FUNCTION_BLOCK FB_SignalHandlingDelay EXTENDS FB_SignalHandling
VAR_INPUT
	tiDelay			: TIME;
END_VAR
VAR
	bSet			: BOOL;
	tonDelay		: TON;
END_VAR

// =========================================================
;
// =========================================================

METHOD PUBLIC M_SetOutput
VAR_INPUT
END_VAR
// =========================================================
	// Out

IF bEnable AND bInput THEN
	bSet := TRUE;
END_IF

IF bSet THEN
	tonDelay(IN := TRUE,
				PT := tiDelay);
ELSE
	tonDelay(IN := FALSE);
END_IF

IF tonDelay.Q THEN
	bSet := FALSE;
	tonDelay(IN := FALSE);
	bOut := TRUE;
ELSE
	bOut := FALSE;
END_IF
			
// =========================================================
END_METHOD

END_FUNCTION_BLOCK
